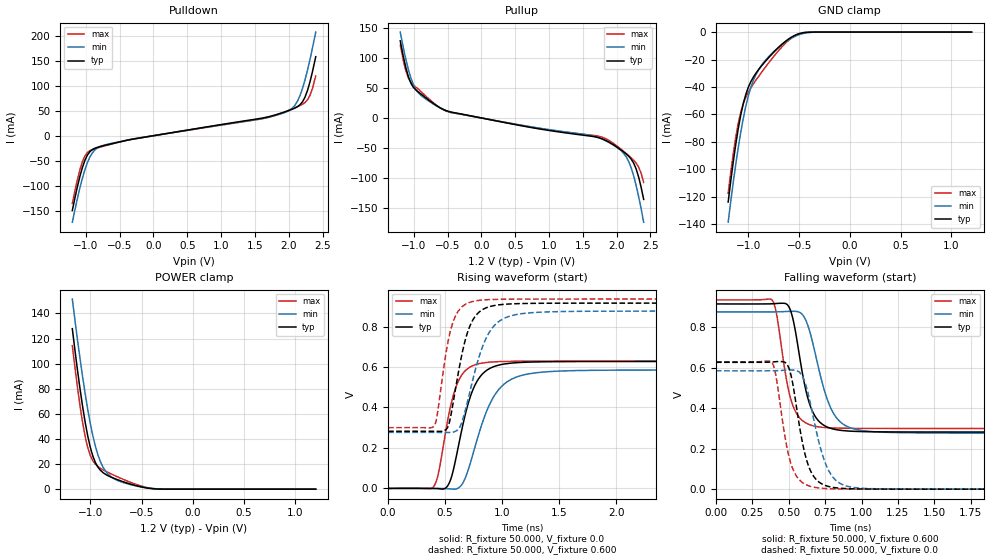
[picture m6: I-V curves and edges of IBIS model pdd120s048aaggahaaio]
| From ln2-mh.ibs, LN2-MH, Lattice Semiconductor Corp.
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|   Model pdd120s048aaggahaaio
[Model] pdd120s048aaggahaaio
| Clamp models do not include dynamic input termination. Please refer to
| the pdd120axxxaaggahaain model for input termination.
Model_type I/O
Polarity   Non-Inverting
Enable   Active-Low
Vinl =  0.800V
Vinh =  1.000V
Vmeas =  0.600V
Cref =  20.000pF
Rref =  50.000
Vref =  0.600V
C_comp   2.000pF   1.500pF   2.500pF
[Temperature Range]   25.000   0.125k   -40.000
[Voltage Range]   1.200V   1.160V   1.240V
[C Comp Corner]
C_comp   2.000pF   1.500pF   2.500pF
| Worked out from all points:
|   slope of the pulldown table from 0 to 0.18 V, typ, clamps not added: 44.5 ohm
|   slope of the pullup table from 0 to 0.18 V, typ, clamps not added: 44.9 ohm
|   GND clamp passes 1 mA (typ) near -0.49 V on its own axis
|   POWER clamp passes 1 mA (typ) near -0.45 V on its own axis
|   rising waveform, R_fixture 50.000, V_fixture 0.0: 20-80 % time 169ps typ, 226ps min, 137ps max; typ from 0 V to 0.627 V
|   rising waveform, R_fixture 50.000, V_fixture 0.600: 20-80 % time 142ps typ, 190ps min, 115ps max; typ from 0.282 V to 0.916 V
|   falling waveform, R_fixture 50.000, V_fixture 0.600: 20-80 % time 105ps typ, 139ps min, 92.4ps max; typ from 0.916 V to 0.282 V
|   falling waveform, R_fixture 50.000, V_fixture 0.0: 20-80 % time 98.6ps typ, 124ps min, 90.5ps max; typ from 0.627 V to 0 V
[Pulldown]
|Voltage   I(typ)   I(min)   I(max)
-1.2V     -149.7mA   -173.1mA   -135.6mA
-1.089V   -81.92mA   -105.1mA   -68.52mA
-1.015V   -49.75mA   -68.65mA   -40.97mA
-904mV    -27.77mA   -34.34mA   -27.75mA
-793mV    -21.85mA   -21.77mA   -23.08mA
-312mV    -7.083mA   -7.064mA   -6.683mA
1.612V    35.31mA    34.52mA    34mA
2.056V    53.27mA    55.43mA    53.91mA
2.167V    61.89mA    80.22mA    60.44mA
2.241V    77.15mA    111.6mA    66.35mA
2.315V    107.9mA    152.7mA    80.79mA
2.4V      158.2mA    207.4mA    119.5mA
[Pullup]
|Voltage   I(typ)   I(min)   I(max)
-1.2V     128.3mA    142.9mA    121.5mA
-1.115V   82.76mA    96.52mA    77.79mA
-1.004V   50.71mA    55.12mA    54.73mA
-893mV    39.8mA     37.51mA    43.84mA
-634mV    18.47mA    18.18mA    18.7mA
-449mV    9.858mA    9.653mA    9.019mA
1.623V    -30.34mA   -29.2mA    -28.61mA
2.03V     -50.48mA   -50.95mA   -48.79mA
2.141V    -59.83mA   -64.48mA   -59mA
2.215V    -68.36mA   -82.83mA   -66.26mA
2.289V    -84.85mA   -112.4mA   -75.03mA
2.4V      -135.5mA   -173.4mA   -107.4mA
[GND_clamp]
|Voltage   I(typ)   I(min)   I(max)
-1.2V     -123.9mA   -138.6mA   -117.5mA
-1.15V    -94.78mA   -109.7mA   -88.79mA
-1.1V     -70.2mA    -84.05mA   -66.33mA
-1.05V    -51.82mA   -62.6mA    -51.98mA
-1.025V   -45.18mA   -53.76mA   -47.32mA
-975mV    -35.96mA   -40.02mA   -40.52mA
-925mV    -29.87mA   -30.81mA   -34.98mA
-875mV    -25.03mA   -24.57mA   -29.81mA
-675mV    -9.229mA   -9.412mA   -11.2mA
-550mV    -2.635mA   -3.442mA   -3.059mA
-425mV    -169.7uA   -547.4uA   -117uA
1.2V      0A         0A         0A
[POWER_clamp]
|Voltage   I(typ)   I(min)   I(max)
-1.175V   127.9mA    151.5mA    114.3mA
-1.125V   95.1mA     119.3mA    81.28mA
-1.1V     80mA       104.2mA    66.46mA
-1.05V    53.45mA    76.25mA    42.06mA
-1.025V   42.52mA    63.79mA    33.25mA
-975mV    26.42mA    42.64mA    22.65mA
-925mV    17.53mA    27.24mA    17.97mA
-875mV    13.15mA    17.46mA    15.37mA
-800mV    9.709mA    10.06mA    12.3mA
-625mV    4.479mA    4.015mA    6.021mA
-350mV    147.7uA    296.5uA    176.7uA
1.2V      0A         0A         0A
[Ramp]
| variable   typ   min   max
dV/dt_r   0.376/0.169n   0.351/0.226n   0.378/0.138n
dV/dt_f   0.380/0.119n   0.365/0.164n   0.383/96.871p
R_load = 50.000
[Rising Waveform]
R_fixture= 50.000
V_fixture= 0.0
V_fixture_min= 0.0
V_fixture_max= 0.0
|time   V(typ)   V(min)   V(max)
0s        1.292uV    7.005uV    589.2nV
397ps     -239uV     71.17uV    7.302mV
442ps     -1.458mV   51.83uV    76.87mV
513ps     6.253mV    -1.073mV   307.5mV
643ps     282mV      16.23mV    558.2mV
742ps     485.9mV    166.3mV    606.6mV
862ps     582.9mV    379.4mV    622.5mV
1.084ns   619.5mV    540.5mV    628.3mV
1.524ns   626.8mV    580.5mV    629.3mV
10ns      627.3mV    585.3mV    629.4mV
[Rising Waveform]
R_fixture= 50.000
V_fixture= 0.600
V_fixture_min= 0.583
V_fixture_max= 0.619
|time   V(typ)   V(min)   V(max)
0s        282.5mV    276.8mV    300.3mV
405ps     282.1mV    276.9mV    309.7mV
514ps     294.8mV    276.3mV    690.4mV
564ps     403.5mV    277.5mV    813.4mV
637ps     635.1mV    313.3mV    891.5mV
712ps     796mV      466.6mV    919mV
804ps     874.5mV    662.3mV    930mV
964ps     906.9mV    822.2mV    934.6mV
1.314ns   915mV      870.6mV    935.9mV
10ns      915.9mV    876.6mV    936mV
[Falling Waveform]
R_fixture= 50.000
V_fixture= 0.600
V_fixture_min= 0.583
V_fixture_max= 0.619
|time   V(typ)   V(min)   V(max)
0s        915.9mV    876.6mV    936mV
386ps     916.6mV    876.7mV    934.6mV
417ps     918.1mV    876.9mV    862.7mV
493ps     910.1mV    878.9mV    508.9mV
535ps     821.4mV    879.4mV    401.6mV
614ps     500.9mV    840.1mV    328.9mV
739ps     316.9mV    502.5mV    305.3mV
869ps     289.9mV    324mV      301.4mV
1.168ns   283.2mV    281.1mV    300.4mV
10ns      282.5mV    276.8mV    300.3mV
[Falling Waveform]
R_fixture= 50.000
V_fixture= 0.0
V_fixture_min= 0.0
V_fixture_max= 0.0
|time   V(typ)   V(min)   V(max)
0s        627.3mV    585.3mV    629.4mV
386ps     628.9mV    585.5mV    624.5mV
487ps     618.4mV    588.7mV    208.5mV
525ps     531.3mV    589mV      105.4mV
603ps     199.9mV    543.9mV    28.35mV
653ps     85.88mV    409.3mV    13.05mV
729ps     25.47mV    176.1mV    4.406mV
839ps     5.581mV    34.81mV    1.117mV
1.063ns   599.6uV    2.461mV    139.9uV
10ns      1.309uV    7.016uV    608.3nV
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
